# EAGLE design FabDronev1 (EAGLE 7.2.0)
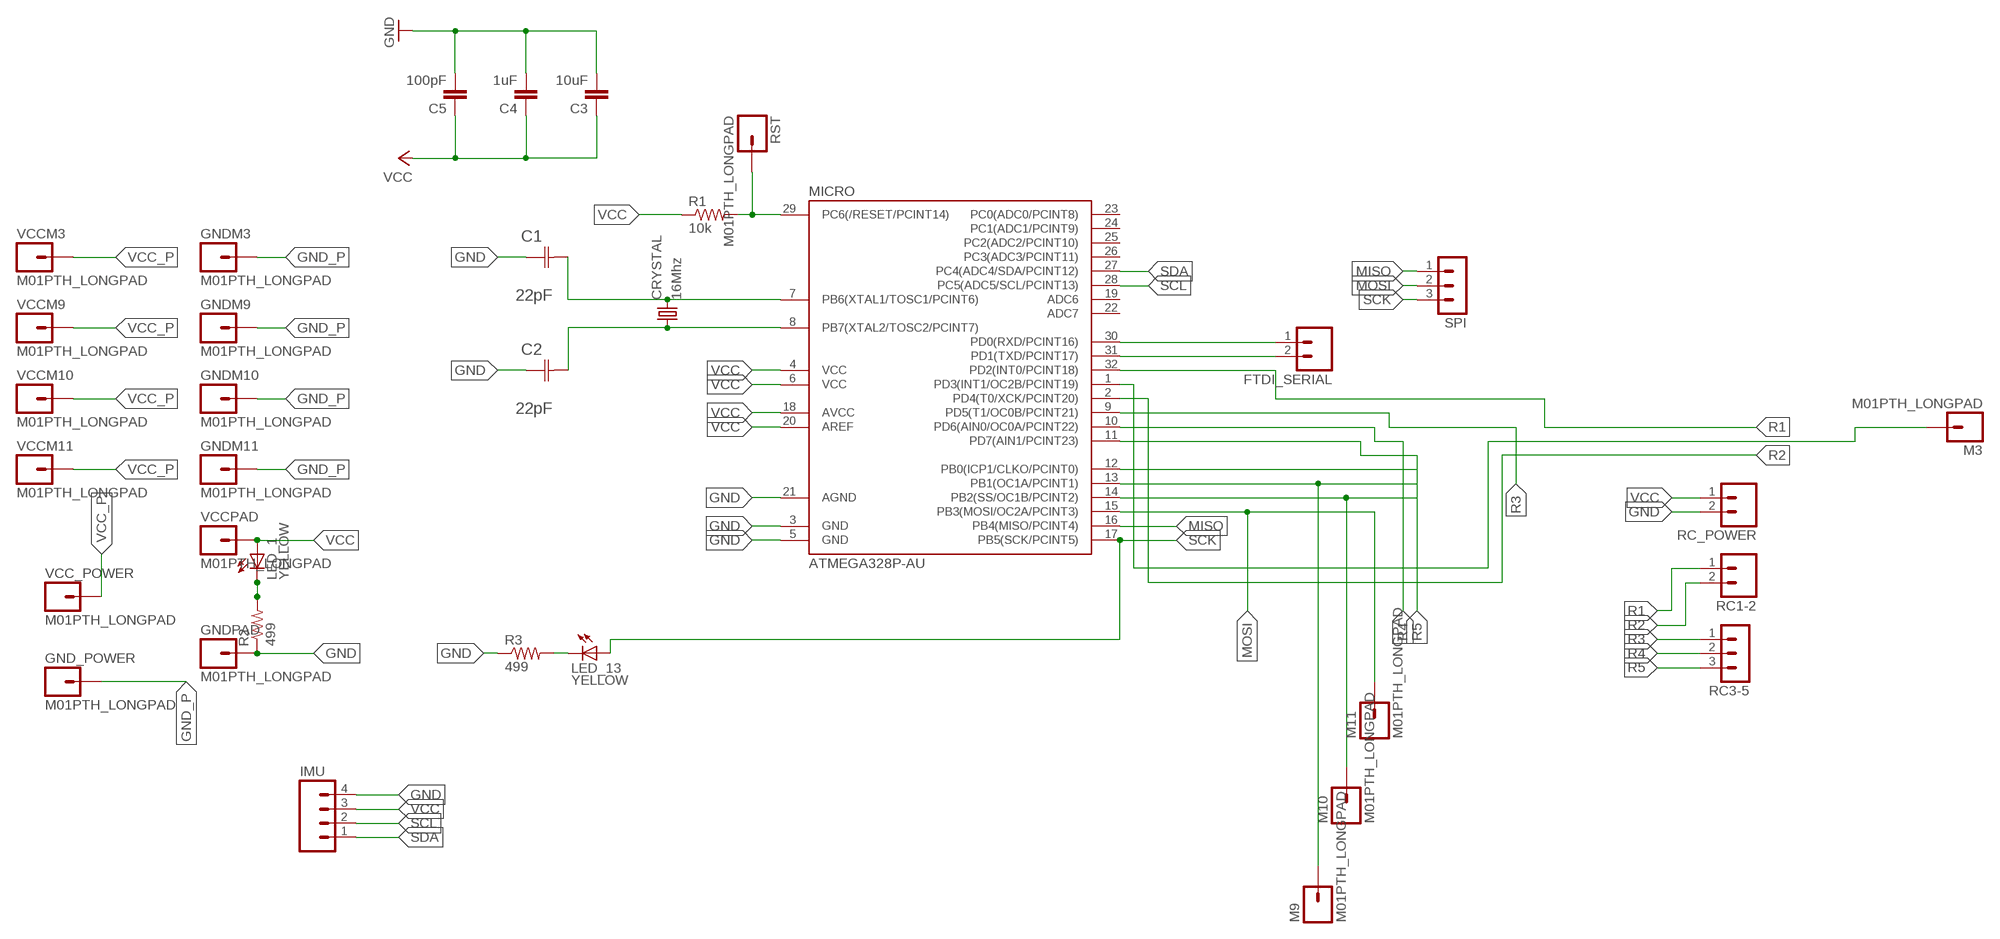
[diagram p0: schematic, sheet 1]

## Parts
C1  22pF  0612ZC225MAT2A  [CAPC3216X178N]
C2  22pF  0612ZC225MAT2A  [CAPC3216X178N]
C3  10uF  CAP1206  [1206]
C4  1uF  CAP1206  [1206]
C5  100pF  CAP1206  [1206]
CRYSTAL  16Mhz  CSM-7X-DU  [CSM-7X-DU]
FTDI_SERIAL  M02LOCK_LONGPADS  [1X02_LOCK_LONGPADS]
GND_POWER  M01PTH_LONGPAD  [1X01_LONGPAD]
GNDM3  M01PTH_LONGPAD  [1X01_LONGPAD]
GNDM9  M01PTH_LONGPAD  [1X01_LONGPAD]
GNDM10  M01PTH_LONGPAD  [1X01_LONGPAD]
GNDM11  M01PTH_LONGPAD  [1X01_LONGPAD]
GNDPAD  M01PTH_LONGPAD  [1X01_LONGPAD]
IMU  M04LONGPADS  [1X04_LONGPADS]
LED_1  YELLOW  LED1206  [1206]
LED_13  YELLOW  LED1206  [1206]
M3  M01PTH_LONGPAD  [1X01_LONGPAD]
M9  M01PTH_LONGPAD  [1X01_LONGPAD]
M10  M01PTH_LONGPAD  [1X01_LONGPAD]
M11  M01PTH_LONGPAD  [1X01_LONGPAD]
MICRO  ATMEGA328P-AU  ATMEGA48/88/168-AU  [TQFP32-08]
R1  10k  RESISTOR1206  [1206]
R2  499  RESISTOR1206  [1206]
R3  499  RESISTOR1206  [1206]
RC1-2  M02  [1X02_LONGPADS]
RC3-5  MA03-1  [MA03-1]
RC_POWER  M02  [1X02_LONGPADS]
RST  M01PTH_LONGPAD  [1X01_LONGPAD]
SPI  MA03-1  [MA03-1]
VCC_POWER  M01PTH_LONGPAD  [1X01_LONGPAD]
VCCM3  M01PTH_LONGPAD  [1X01_LONGPAD]
VCCM9  M01PTH_LONGPAD  [1X01_LONGPAD]
VCCM10  M01PTH_LONGPAD  [1X01_LONGPAD]
VCCM11  M01PTH_LONGPAD  [1X01_LONGPAD]
VCCPAD  M01PTH_LONGPAD  [1X01_LONGPAD]

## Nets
GND: C1.1(C1) C2.1(C1) C3.2 C4.2 C5.2 GNDPAD.1 IMU.4 MICRO.3(GND) MICRO.5(GND) MICRO.21(AGND) R2.1 R3.1 RC_POWER.2
GND_P: GND_POWER.1 GNDM3.1 GNDM9.1 GNDM10.1 GNDM11.1
MISO: MICRO.16(PB4(MISO/PCINT4)) SPI.1
MOSI: M11.1 MICRO.15(PB3(MOSI/OC2A/PCINT3)) SPI.2
N$1: LED_1.2(C) R2.2
N$2: C1.2(C2) CRYSTAL.2 MICRO.7(PB6(XTAL1/TOSC1/PCINT6))
N$3: MICRO.29(PC6(/RESET/PCINT14)) R1.2 RST.1
N$6: MICRO.12(PB0(ICP1/CLKO/PCINT0))
N$7: M9.1 MICRO.13(PB1(OC1A/PCINT1))
N$8: M10.1 MICRO.14(PB2(SS/OC1B/PCINT2))
N$9: C2.2(C2) CRYSTAL.1 MICRO.8(PB7(XTAL2/TOSC2/PCINT7))
N$13: FTDI_SERIAL.1 MICRO.30(PD0(RXD/PCINT16))
N$19: FTDI_SERIAL.2 MICRO.31(PD1(TXD/PCINT17))
N$23: M3.1 MICRO.1(PD3(INT1/OC2B/PCINT19))
N$27: LED_13.2(C) R3.2
R1: MICRO.32(PD2(INT0/PCINT18)) RC1-2.1
R2: MICRO.2(PD4(T0/XCK/PCINT20)) RC1-2.2
R3: MICRO.9(PD5(T1/OC0B/PCINT21)) RC3-5.1
R4: MICRO.10(PD6(AIN0/OC0A/PCINT22)) RC3-5.2
R5: MICRO.11(PD7(AIN1/PCINT23)) RC3-5.3
SCK: LED_13.1(A) MICRO.17(PB5(SCK/PCINT5)) SPI.3
SCL: IMU.2 MICRO.28(PC5(ADC5/SCL/PCINT13))
SDA: IMU.1 MICRO.27(PC4(ADC4/SDA/PCINT12))
VCC: C3.1 C4.1 C5.1 IMU.3 LED_1.1(A) MICRO.4(VCC) MICRO.6(VCC) MICRO.18(AVCC) MICRO.20(AREF) R1.1 RC_POWER.1 VCCPAD.1
VCC_P: VCC_POWER.1 VCCM3.1 VCCM9.1 VCCM10.1 VCCM11.1
Unconnected: MICRO.19(ADC6) MICRO.22(ADC7) MICRO.23(PC0(ADC0/PCINT8)) MICRO.24(PC1(ADC1/PCINT9)) MICRO.25(PC2(ADC2/PCINT10)) MICRO.26(PC3(ADC3/PCINT11))

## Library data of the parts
C1 C2 = AVX_By_element14_Batch_1:0612ZC225MAT2A: Capacitor 1206; MPN: 0612ZC225MAT2A; OC_FARNELL: -; OC_NEWARK: 12N3209; SUPPLIER: AVX; TOLERANCE: ±20%; VALUE: 2.2µF; VOLTAGERATING: 10V
C3-C5 = 01_SparkFun:CAP: Capacitor
CRYSTAL = 01_FAB_Hello:CSM-7X-DU: SMD CRYSTAL; OC_FARNELL: unknown; OC_NEWARK: unknown
FTDI_SERIAL RC1-2 RC_POWER = 01_SparkFun:M02: Header 2
GND_POWER GNDM3 GNDM9-GNDM11 GNDPAD M3 M9-M11 RST VCC_POWER VCCM3 VCCM9-VCCM11 VCCPAD = 01_SparkFun:M01: Header 1
IMU = 01_SparkFun:M04: Header 4 Standard 4-pin 0.1" header. Use with straight break away headers (SKU : PRT-00116), right angle break away headers (PRT-00553), swiss pins (PRT-00743), machine pins (PRT-00117), and female headers (PRT-00115). Molex polarized connector foot print use with SKU : PRT-08231 with associated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
LED_1 LED_13 = 01_FAB_Hello:LED
MICRO = atmega8:ATMEGA48/88/168
R1-R3 = 01_SparkFun:RESISTOR: Resistor
RC3-5 SPI = con-lstb:MA03-1: PIN HEADER; OC_FARNELL: unknown; OC_NEWARK: unknown

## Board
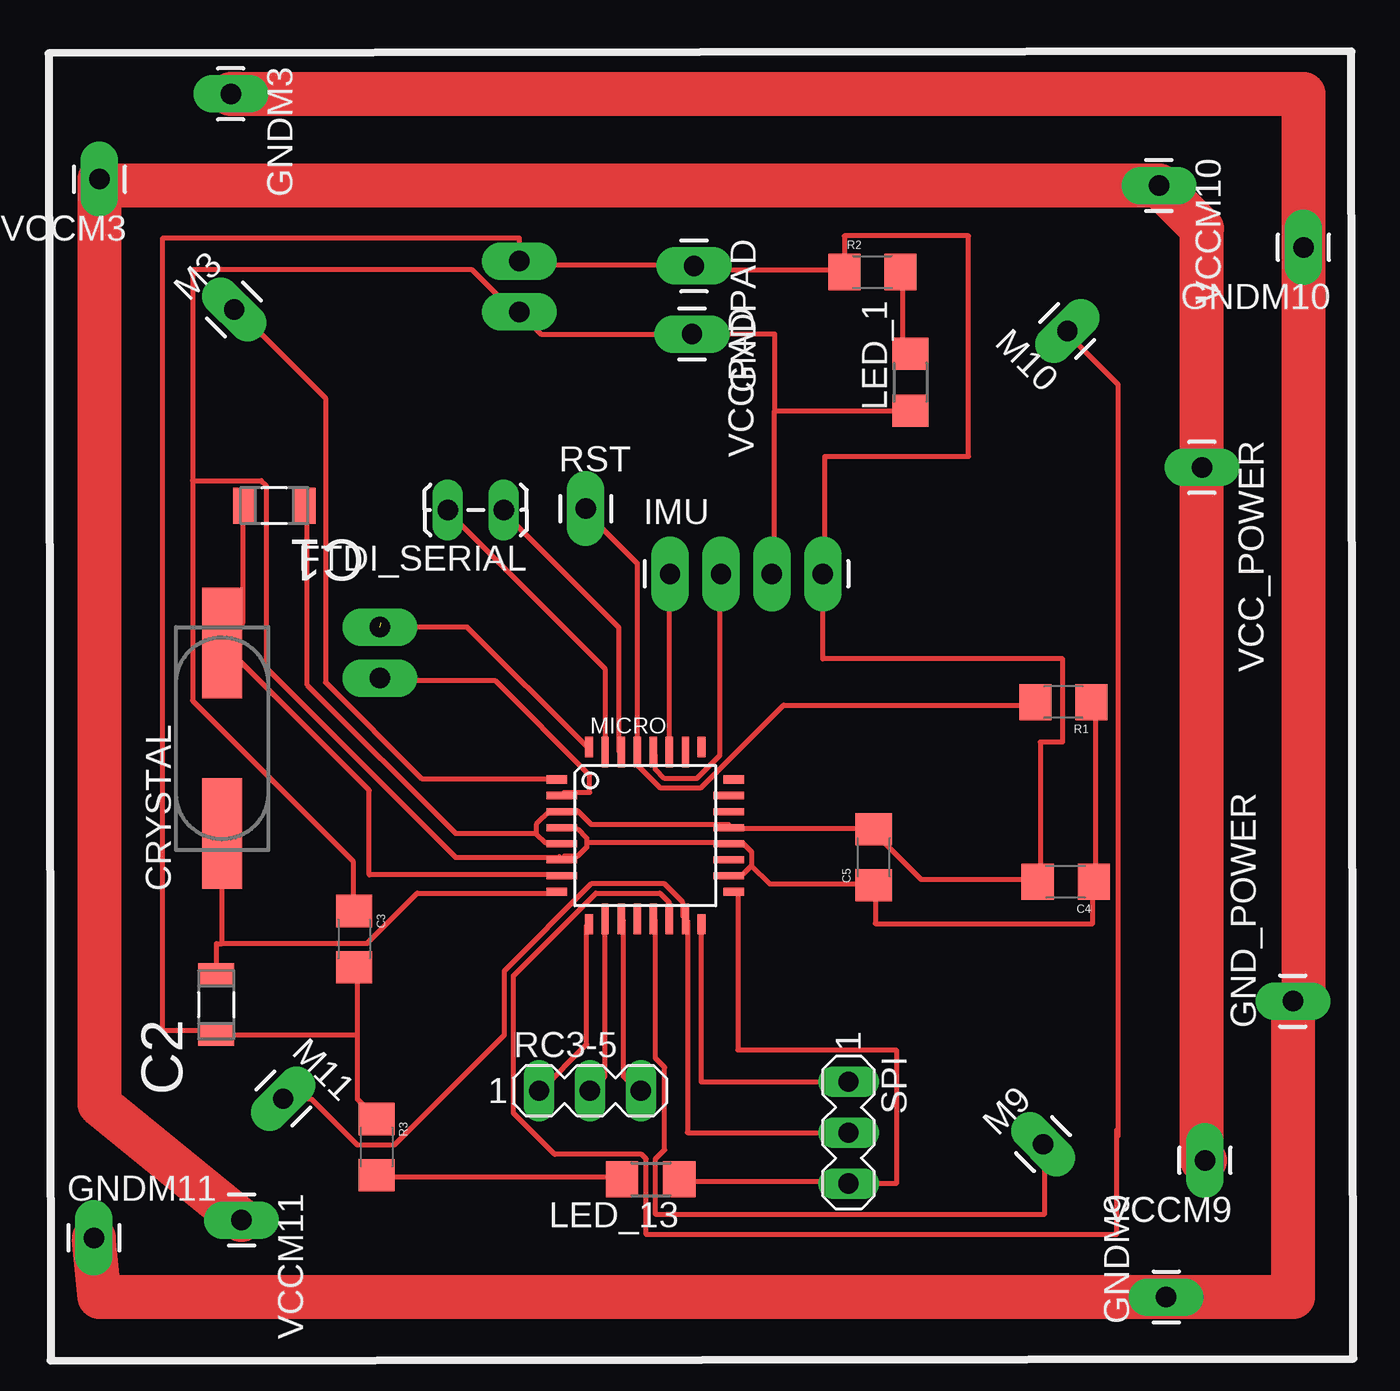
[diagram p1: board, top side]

No outline drawn. Coordinates in mm, seen from the top.
Copper layers (1*16): Top 0.035mm / dielectric 1.5mm / Bottom 0.035mm
Design rules "default": minimum track width 10mil, minimum drill 24mil, track to track 8mil, track to pad 8mil, pad to pad 8mil, via to via 8mil, smd to smd 8mil, copper to edge 40mil, drill to drill 8mil, minimum pad ring 10mil, minimum via ring 8mil, stop-mask expansion 4mil, vias tented up to drill 0mil, thermal gap 10mil

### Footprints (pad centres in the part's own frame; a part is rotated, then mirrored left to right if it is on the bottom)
CAPC3216X178N = smd 1.118 x 1.803: 1 -1.499,0; 2 1.499,0
1206 = smd 1.6 x 1.8: 1 -1.4,0; 2 1.4,0
CSM-7X-DU = smd 5.5 x 2: 1 -4.75,0; 2 4.75,0
1X02_LOCK_LONGPADS = drill 1.016 long: 1 -0.127,0; 2 2.667,0
1X01_LONGPAD = drill 1.016 pad 1.88 long: 1 0,0
1X04_LONGPADS = drill 1.016 pad 1.88 long: 1 0,0; 2 2.54,0; 3 5.08,0; 4 7.62,0
1206' = smd 1.6 x 1.803: 1 -1.422,0; 2 1.422,0
TQFP32-08 = smd 1.016 x 0.406: 1 -4.42,2.8; 8 -4.42,-2.8; 17 4.42,-2.8; 24 4.42,2.8 | smd 1.524 x 0.356: 2 -4.166,2; 3 -4.166,1.2; 4 -4.166,0.4; 5 -4.166,-0.4; 6 -4.166,-1.2; 7 -4.166,-2; 18 4.166,-2; 19 4.166,-1.2; 20 4.166,-0.4; 21 4.166,0.4; 22 4.166,1.2; 23 4.166,2 | smd 0.406 x 1.016: 9 -2.8,-4.42; 16 2.8,-4.42; 25 2.8,4.42; 32 -2.8,4.42 | smd 0.356 x 1.524: 10 -2,-4.166; 11 -1.2,-4.166; 12 -0.4,-4.166; 13 0.4,-4.166; 14 1.2,-4.166; 15 2,-4.166; 26 2,4.166; 27 1.2,4.166; 28 0.4,4.166; 29 -0.4,4.166; 30 -1.2,4.166; 31 -2,4.166
1X02_LONGPADS = drill 1.016 pad 1.88 long: 1 0,0; 2 2.54,0
MA03-1 = drill 1.016 long: 1 -2.54,0; 2 0,0; 3 2.54,0

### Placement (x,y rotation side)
C1  11.16,42.65 180 top
C2  8.27,17.75 90 top
C3  15.15,21.03 270 top
C4  50.65,23.87 180 top
C5  41.07,25.1 90 top
CRYSTAL  8.56,31.04 90 top
FTDI_SERIAL  22.48,42.43 180 top
GND_POWER  61.99,17.93 90 top
GNDM3  8.99,63.18 270 top
GNDM9  55.67,3.17 90 top
GNDM10  62.51,55.53 180 top
GNDM11  2.16,6.12 0 top
GNDPAD  32.1,54.6 270 top
IMU  30.91,39.24 0 top
LED_1  YELLOW  [1206']  42.9,48.8 90 top
LED_13  YELLOW  [1206']  29.94,9.04 180 top
M3  9.16,52.42 45 top
M9  49.52,10.79 45 top
M10  50.73,51.36 135 top
M11  11.6,13.06 315 top
MICRO  29.67,26.18 0 top
R1  50.53,32.84 180 top
R2  41,54.3 0 top
R3  16.26,10.65 270 top
RC1-2  16.43,36.59 270 top
RC3-5  26.91,13.46 0 top
RC_POWER  23.38,52.31 90 top
RST  26.7,42.5 0 top
SPI  39.81,11.37 270 top
VCC_POWER  57.45,44.55 270 top
VCCM3  2.44,58.94 180 top
VCCM9  57.6,9.99 180 top
VCCM10  55.31,58.61 270 top
VCCM11  9.52,7 270 top
VCCPAD  32,51.2 270 top

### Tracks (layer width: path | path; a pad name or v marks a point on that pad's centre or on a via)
GND
  Top 0.254: 24.23,26.29 24.69,25.83 25.38,25.83 MICRO.5 | 24.23,26.29 24.23,26.75 24.92,27.43 25.38,27.43 MICRO.3 25.6,27.43 26.29,27.43 26.98,26.75 33.83,26.75 MICRO.21 34.06,26.52 40.92,26.52 C5.2 41.15,26.29 43.43,24 49.15,24 C4.2 49.38,24 49.38,30.86 50.5,30.86 50.5,35 38.53,35 IMU.4 38.63,39.32 38.63,45.1 45.8,45.1 45.8,56.1 39.6,56.1 R2.1 | C1.1 12.8,42.52 12.8,33.7 20.2,26.3 24.22,26.3 24.23,26.29 | 15.32,16.23 15.32,13.03 16.23,12.12 R3.1 | 15.32,16.23 15.32,19.43 C3.2 | 15.32,16.23 8.46,16.23 C2.1 8.23,16.46 5.6,16.46 5.6,56 23.38,56 RC_POWER.2 | R2.1 39.55,54.41 32.23,54.41 GNDPAD.1 32,54.63 23.55,54.63 RC_POWER.2 | 39.78,54.18 R2.1 | 23.32,54.86 RC_POWER.2
GND_P
  Top 2.184: GNDM3.1 62.51,63.18 GNDM10.1 62.51,18.46 GND_POWER.1 61.99,3.17 GNDM9.1 2.44,3.17 GNDM11.1
MISO
  Top 0.254: MICRO.16 32.46,21.72 32.46,13.91 SPI.1 39.78,13.95
MOSI
  Top 0.254: 39.78,11.43 SPI.2 31.77,11.37 31.77,21.95 MICRO.15 31.55,22.17 31.55,22.86 30.63,23.77 26.98,23.77 22.63,19.43 22.63,16.23 17.14,10.74 15.32,10.74 13.03,13.03 11.66,13.03 M11.1
N$1
  Top 0.254: R2.2 42.52,54.18 42.52,50.52 42.75,50.29 LED_1.2
N$2
  Top 0.254: MICRO.7 25.38,24.23 15.9,24.23 15.9,28.45 CRYSTAL.2 | 8.69,35.66 CRYSTAL.2 | C1.2 9.6,42.52 9.6,36.8 8.69,35.89 CRYSTAL.2
N$3
  Top 0.254: RST.1 26.75,42.29 29.26,39.78 29.26,30.4 MICRO.29 29.26,30.18 29.26,29.72 30.4,28.57 32.46,28.57 36.58,32.69 48.92,32.69 R1.2
N$7
  Top 0.254: MICRO.13 30.18,21.95 30.18,15.09 30.63,14.63 30.63,10.52 30.18,10.06 30.18,7.3 49.6,7.3 49.6,10.79 M9.1 49.38,10.74
N$8
  Top 0.254: 53.26,11.5 53.26,48.69 50.75,51.21 M10.1 | 53.26,11.5 53.26,11.2 | MICRO.14 30.86,22.17 30.86,22.86 30.4,23.32 27.2,23.32 23.09,19.2 23.09,12.34 25.15,10.29 29.49,10.29 29.72,10.06 29.72,6.3 53.2,6.3 53.2,11.5 53.26,11.5
N$9
  Top 0.254: MICRO.8 25.15,23.32 18.29,23.32 15.77,20.8 8.56,20.8 | 8.46,19.43 C2.2 8.27,20.8 8.56,20.8 | 8.69,26.29 CRYSTAL.1 8.56,20.8
N$13
  Top 0.254: MICRO.30 28.35,30.4 28.35,36.58 22.63,42.29 FTDI_SERIAL.1
N$19
  Top 0.254: MICRO.31 27.66,30.4 27.66,34.52 19.89,42.29 FTDI_SERIAL.2
N$23
  Top 0.254: MICRO.1 25.15,29.03 18.52,29.03 13.72,33.83 13.72,48.01 9.37,52.35 M3.1
N$27
  Top 0.254: R3.2 16.46,9.14 28.35,9.14 LED_13.2
R1  (1 unrouted)
  Top 0.254: MICRO.32 26.75,30.63 20.79,36.59 RC1-2.1
R2
  Top 0.254: MICRO.2 25.6,28.35 26.9,28.35 26.9,29.2 22.2,33.9 16.57,33.9 RC1-2.2
R3
  Top 0.254: MICRO.9 26.75,21.72 26.75,15.77 24.46,13.49 RC3-5.1
R4
  Top 0.254: MICRO.10 27.66,21.95 27.66,14.17 26.98,13.49 RC3-5.2
R5
  Top 0.254: MICRO.11 28.57,21.95 28.57,14.17 29.26,13.49 RC3-5.3
SCK
  Top 0.254: MICRO.17 34.29,23.32 34.29,15.5 42.2,15.5 42.2,8.83 SPI.3 | 40.01,8.91 SPI.3 | LED_13.1 31.55,8.91 39.78,8.91 SPI.3
SCL
  Top 0.254: MICRO.28 30.18,30.18 30.18,29.49 30.63,29.03 32.23,29.03 33.38,30.18 33.38,39.09 IMU.2
SDA
  Top 0.254: MICRO.27 30.86,30.4 30.86,39.09 IMU.1
VCC
  Top 0.254: C4.1 52.12,24 52.12,32.69 R1.1 | 26.75,25.83 26.75,26.06 26.29,26.52 25.6,26.52 MICRO.4 | 26.75,25.83 26.75,25.6 26.29,25.15 25.6,25.15 MICRO.6 | 34.98,24.69 34.52,24.23 34.06,24.23 MICRO.18 | 34.98,24.69 34.98,25.38 34.52,25.83 34.06,25.83 MICRO.20 33.83,25.83 26.75,25.83 | 34.98,24.69 35.89,23.77 40.92,23.77 C5.1 41.15,23.55 41.15,21.8 52,21.8 52,23.88 C4.1 | 51.44,23.77 51.89,23.77 C4.1 | IMU.3 36.12,39.32 36.12,47.38 | 7.09,43.89 7.09,54.41 21.03,54.41 23.32,52.12 RC_POWER.1 23.55,52.12 24.46,51.21 31.77,51.21 VCCPAD.1 | 7.09,43.89 7.09,32.92 15.09,24.92 15.09,22.63 C3.1 | 31.77,50.98 VCCPAD.1 | 7.09,43.89 10.52,43.89 10.74,43.66 10.74,34.56 20.2,25.1 25.39,25.1 MICRO.6 | 25.38,25.15 MICRO.6 | VCCPAD.1 36.12,51.2 36.12,47.38 | 36.12,47.38 LED_1.1
VCC_P
  Top 2.184: VCCM9.1 57.45,9.98 VCC_POWER.1 57.45,56.47 VCCM10.1 2.76,58.61 VCCM3.1 2.44,12.79 VCCM11.1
